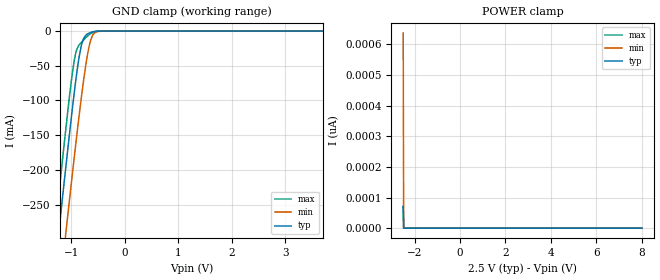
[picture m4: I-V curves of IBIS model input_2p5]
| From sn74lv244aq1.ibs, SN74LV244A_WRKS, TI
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[Model]   input_2p5
Model_type   Input
Vinl = 0.75
Vinh = 1.75
|   typ   min   max
C_comp   2.237pF   2.216pF   2.352pF
[Voltage Range]   2.5   2.3   2.7
[Temperature Range]   25   125   -40
[Power Clamp Reference]   2.5   2.3   2.7
[GND Clamp Reference]   0   0   0
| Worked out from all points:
|   GND clamp passes 1 mA (typ) near -0.59 V on its own axis
[GND Clamp]
|   Voltage   I(typ)   I(min)   I(max)
-2.5V     -1.244A    -1.327A    -1.203A
-1.313V   -350.3mA   -444.6mA   -296.5mA
-1.23V    -289mA     -383.9mA   -234.5mA
-1.125V   -213.4mA   -308.8mA   -158.5mA
-1.072V   -176.4mA   -271.7mA   -121.6mA
-977.5mV  -111.7mA   -206mA     -60.6mA
-914.5mV  -71.44mA   -163.3mA   -31.85mA
-799mV    -17.49mA   -89.06mA   -15.38mA
-704.5mV  -4.594mA   -38.07mA   -7.858mA
-631mV    -1.797mA   -12.21mA   -3.542mA
-442mV    -17.94uA   -111.5uA   -18.13uA
8V        0A         0A         0A
[POWER Clamp]
|   Voltage   I(typ)   I(min)   I(max)
-2.5V     69.79pA    637.9pA    71.28pA
-2.479V   0A         0A         0A
-1mV      0A         0A         0A
8V        0A         0A         0A
